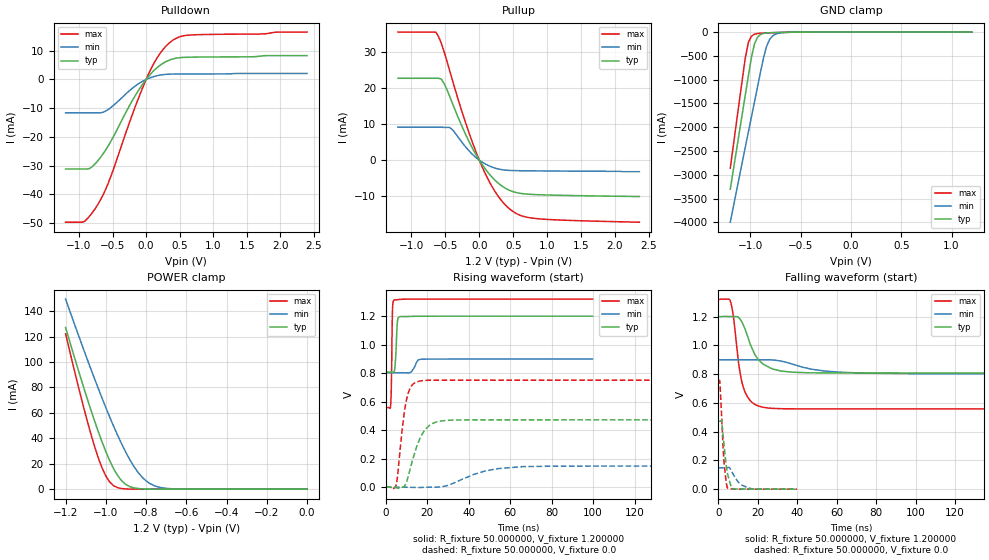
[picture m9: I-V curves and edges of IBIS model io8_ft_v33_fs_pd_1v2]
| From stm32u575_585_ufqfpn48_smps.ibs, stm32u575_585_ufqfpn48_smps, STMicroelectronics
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|   Model io8_ft_v33_fs_pd_1v2
[Model]  io8_ft_v33_fs_pd_1v2
Model_type I/O
Polarity   Non-Inverting
Enable   Active-Low
Vinl =   0.360000V
Vinh =   0.840000V
Vmeas =  0.600000V
Cref =   50.000000pF
Rref =   100.000000M
Vref =   0.0V
C_comp   2.887200pF   2.816900pF   2.935200pF
[Temperature Range]   25.000000   0.140000k   -40.000000
[Pullup Reference]   1.200000V   0.900000V   1.320000V
[Pulldown Reference]   0.0V   0.0V   0.0V
[POWER Clamp Reference]   1.200000V   0.900000V   1.320000V
[GND Clamp Reference]   0.0V   0.0V   0.0V
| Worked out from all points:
|   slope of the pulldown table from 0 to 0.18 V, typ, clamps not added: 40.7 ohm
|   slope of the pullup table from 0 to 0.18 V, typ, clamps not added: 39.5 ohm
|   GND clamp passes 1 mA (typ) near -0.51 V on its own axis
|   POWER clamp passes 1 mA (typ) near -0.86 V on its own axis
|   rising waveform, R_fixture 50.000000, V_fixture 1.200000: 20-80 % time 758ps typ, 2.06ns min, 446ps max; typ from 0.808 V to 1.2 V
|   rising waveform, R_fixture 50.000000, V_fixture 0.0: 20-80 % time 6.65ns typ, 16.9ns min, 3.63ns max; typ from 0 V to 0.472 V
|   falling waveform, R_fixture 50.000000, V_fixture 1.200000: 20-80 % time 8.06ns typ, 18.7ns min, 4.69ns max; typ from 1.2 V to 0.808 V
|   falling waveform, R_fixture 50.000000, V_fixture 0.0: 20-80 % time 2.49ns typ, 4.75ns min, 1.84ns max; typ from 0.472 V to 0 V
[Pulldown]
|Voltage   I(typ)   I(min)   I(max)
-1.2V     -31.16mA   -11.61mA   -49.71mA
-920mV    -31.16mA   -11.61mA   -49.48mA
-840mV    -31mA      -11.61mA   -47.54mA
-720mV    -28.33mA   -11.61mA   -43.58mA
-560mV    -22.95mA   -10.37mA   -35.89mA
-200mV    -7.146mA   -2.964mA   -11.89mA
0V        0A         0A         -10fA
160mV     4.047mA    1.298mA    7.361mA
360mV     6.87mA     1.87mA     13mA
480mV     7.543mA    1.91mA     14.69mA
640mV     7.765mA    1.923mA    15.46mA
2.4V      8.316mA    2.102mA    16.52mA
[Pullup]
|Voltage   I(typ)   I(min)   I(max)
-1.2V     22.75mA    9.163mA    35.58mA
-640mV    22.75mA    9.163mA    35.53mA
-560mV    22.49mA    9.163mA    32.42mA
-520mV    21.33mA    9.097mA    30.17mA
-400mV    15.99mA    8.534mA    22.45mA
-200mV    7.069mA    3.642mA    10.26mA
40mV      -1.16mA    -508.1uA   -1.774mA
240mV     -5.73mA    -2.256mA   -8.953mA
480mV     -8.639mA   -2.877mA   -14.04mA
640mV     -9.31mA    -2.942mA   -15.55mA
880mV     -9.601mA   -2.986mA   -16.29mA
2.36V     -10.1mA    -3.2mA     -17.23mA
[GND_clamp]
|Voltage   I(typ)   I(min)   I(max)
-1.2V     -3.305A    -3.998A    -2.862A
-1.05V    -1.316A    -2.418A    -539.3mA
-1.02V    -921mA     -2.103A    -218.8mA
-990mV    -539.5mA   -1.788A    -87.45mA
-960mV    -252.2mA   -1.474A    -44.37mA
-930mV    -110.5mA   -1.16A     -30.33mA
-870mV    -28.04mA   -549.1mA   -21.1mA
-840mV    -18.44mA   -305.6mA   -18.29mA
-810mV    -13.92mA   -159.7mA   -15.75mA
-780mV    -11.24mA   -82.36mA   -13.39mA
-600mV    -2.986mA   -4.279mA   -3.072mA
1.2V      30.28uA    18.17uA    37.27uA
[POWER_clamp]
|Voltage   I(typ)   I(min)   I(max)
-1.2V     127mA      149.4mA    122.2mA
-1.12V    84.97mA    114mA      70.27mA
-1.06V    55.51mA    88.42mA    35.67mA
-1.02V    37.63mA    72.04mA    17.17mA
-1V       29.51mA    64.13mA    10.3mA
-960mV    15.69mA    48.99mA    2.571mA
-900mV    3.624mA    28.77mA    182.8uA
-840mV    490.7uA    13.24mA    11.35uA
-800mV    116.8uA    6.532mA    1.77uA
-740mV    13.2uA     1.723mA    109.1nA
-620mV    167.3nA    79.35uA    0A
0V        0A         17.84nA    0A
[Ramp]
| variable   typ   min   max
dV/dt_r  0.28340/6.64217n   88.84188m/16.85636n 0.45045/3.62320n
dV/dt_f  0.23488/8.04595n   58.05000m/18.66238n 0.45673/4.67859n
R_load = 50.000000
[Rising Waveform]
R_fixture= 50.000000
V_fixture= 1.200000
V_fixture_min= 0.900000
V_fixture_max= 1.320000
|time   V(typ)   V(min)   V(max)
0s        808mV      802.7mV    558.2mV
2.402ns   808.1mV    802.7mV    591.8mV
2.603ns   808mV      802.7mV    676.4mV
3.203ns   806.6mV    802.7mV    1.252V
4.204ns   820.9mV    802.7mV    1.314V
5.606ns   1.167V     802.7mV    1.315V
6.607ns   1.195V     802.7mV    1.317V
11.81ns   1.198V     804.9mV    1.319V
17.02ns   1.199V     897.2mV    1.319V
99.7ns    1.199V     899.4mV    1.319V
[Rising Waveform]
R_fixture= 50.000000
V_fixture= 0.0
V_fixture_min= 0.0
V_fixture_max= 0.0
|time   V(typ)   V(min)   V(max)
0s        7.318uV    -73.19nV   9.967uV
4.805ns   -2.708mV   1.399uV    6.197mV
8.008ns   -369.3uV   6.65uV     422.9mV
10.01ns   38.86mV    46.94uV    617.5mV
12.41ns   165mV      -870.9uV   711.2mV
16.42ns   341.6mV    -2.088mV   745mV
21.22ns   436.5mV    -44.74uV   750.3mV
30.43ns   469.5mV    16.05mV    750.6mV
65.67ns   472.3mV    144mV      750.7mV
199.4ns   472.3mV    148.1mV    750.7mV
[Falling Waveform]
R_fixture= 50.000000
V_fixture= 1.200000
V_fixture_min= 0.900000
V_fixture_max= 1.320000
|time   V(typ)   V(min)   V(max)
0s        1.199V     899.4mV    1.319V
6.006ns   1.2V       899.8mV    1.314V
7.608ns   1.201V     900mV      1.211V
10.41ns   1.194V     900mV      868.9mV
12.41ns   1.152V     899.8mV    723.4mV
16.02ns   1.017V     899.6mV    619.6mV
21.22ns   889.1mV    899.6mV    574.7mV
31.63ns   822.2mV    890.8mV    559.5mV
46.05ns   809mV      837.9mV    558.2mV
199.4ns   808mV      802.7mV    558.2mV
[Falling Waveform]
R_fixture= 50.000000
V_fixture= 0.0
V_fixture_min= 0.0
V_fixture_max= 0.0
|time   V(typ)   V(min)   V(max)
0s        472.3mV    148.1mV    750.7mV
800.8ps   472.1mV    148.1mV    747.8mV
1.762ns   470.9mV    148.1mV    500.9mV
2.963ns   307.4mV    148.1mV    188.7mV
4.164ns   155.6mV    148mV      38.15mV
4.885ns   98.98mV    149.8mV    5.628mV
7.447ns   3.719mV    108.2mV    1.314mV
10.89ns   1.133mV    39.02mV    367.5uV
15.3ns    405.5uV    8.836mV    128.2uV
39.88ns   7.318uV    -73.19nV   9.967uV
